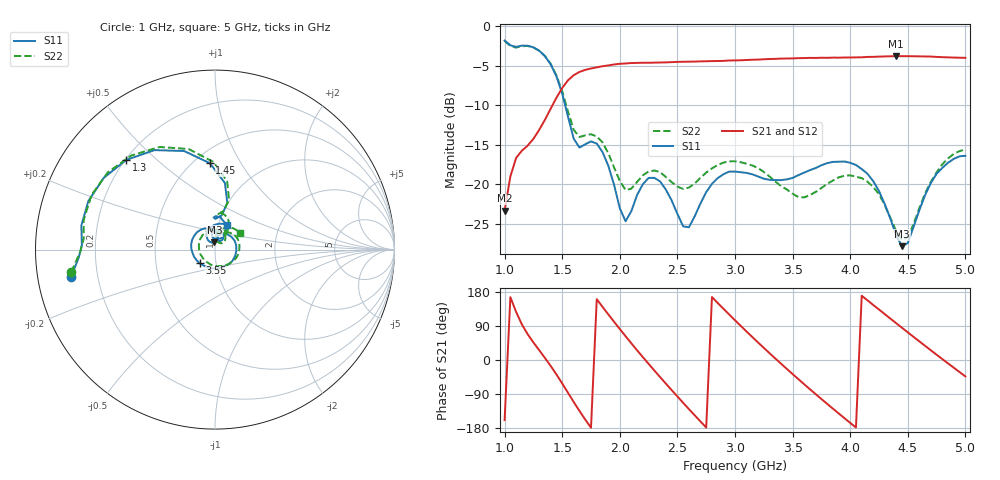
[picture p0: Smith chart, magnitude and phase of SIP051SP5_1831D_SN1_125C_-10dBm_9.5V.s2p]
# GHz  S  dB  R  50
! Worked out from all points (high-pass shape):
!   81 points, 1 GHz to 5 GHz, reference 50 ohm
!   highest |S21| = -3.76 dB at 4.4 GHz (marker M1); lowest = -23.4 dB at 1 GHz (marker M2)
!   |S21| within 3 dB of the highest: 1.555 GHz to end of sweep
!   lowest |S11| = -27.9 dB at 4.45 GHz (marker M3), VSWR 1.08, Z = 49.5 + j4.01 ohm
!   |S11| at or under -10 dB: 1.526 GHz to end of sweep
!   |S22| runs from -27.1 to -1.8 dB; largest |S21 - S12| = 0.0027
!   S11 on the Smith chart (normalised r, x): 1 GHz: 0.10, -0.09; 1.3 GHz: 0.20, +0.40; 1.45 GHz: 0.59, +0.75; 3.55 GHz: 0.83, -0.13; 5 GHz: 1.10, +0.31
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1  -1.77 -169.3  -23.37 -158.7  -23.37 -158.9  -1.82 -171.1
1.1  -2.59 178.0  -16.66 126.7  -16.71 126.8  -2.68 175.4
1.3  -3.06 134.7  -13.11 26.0  -13.13 26.1  -3.08 131.7
1.45  -6.33 93.4  -9.03 -38.1  -9.03 -38.2  -6.21 91.2
1.6  -14.24 79.1  -6.17 -110.8  -6.16 -110.8  -13.10 77.3
1.7  -14.93 92.6  -5.50 -157.1  -5.50 -157.1  -13.80 85.9
1.85  -15.92 70.2  -5.04 140.2  -5.04 140.3  -14.71 66.4
2  -23.05 63.0  -4.73 81.8  -4.73 81.8  -19.59 59.6
2.2  -20.00 96.2  -4.60 7.6  -4.61 7.7  -18.87 77.2
2.35  -19.65 68.5  -4.57 -45.2  -4.56 -45.1  -18.47 61.4
2.5  -23.76 53.1  -4.49 -96.3  -4.50 -96.3  -20.30 53.9
2.7  -22.44 76.9  -4.42 -162.1  -4.41 -162.2  -19.18 57.2
3  -18.39 11.4  -4.30 104.9  -4.29 104.8  -17.09 16.6
3.3  -19.45 -75.0  -4.12 17.9  -4.13 17.9  -19.02 -44.4
3.55  -18.85 -138.3  -4.01 -50.5  -4.01 -50.5  -21.63 -123.5
3.7  -17.95 -171.3  -3.99 -90.0  -3.98 -90.0  -20.98 178.8
4.05  -17.56 117.2  -3.92 -178.2  -3.90 -178.2  -19.04 82.9
4.35  -24.39 75.9  -3.78 109.0  -3.80 109.1  -24.31 40.7
4.4  -26.56 79.3  -3.76 96.9  -3.76 96.9  -25.95 43.9
4.45  -27.86 94.3  -3.77 84.9  -3.75 85.0  -27.07 56.7
4.75  -18.68 109.6  -3.86 13.9  -3.87 14.0  -18.49 72.9
5  -16.40 63.7  -3.97 -43.4  -3.99 -43.4  -15.59 33.5
